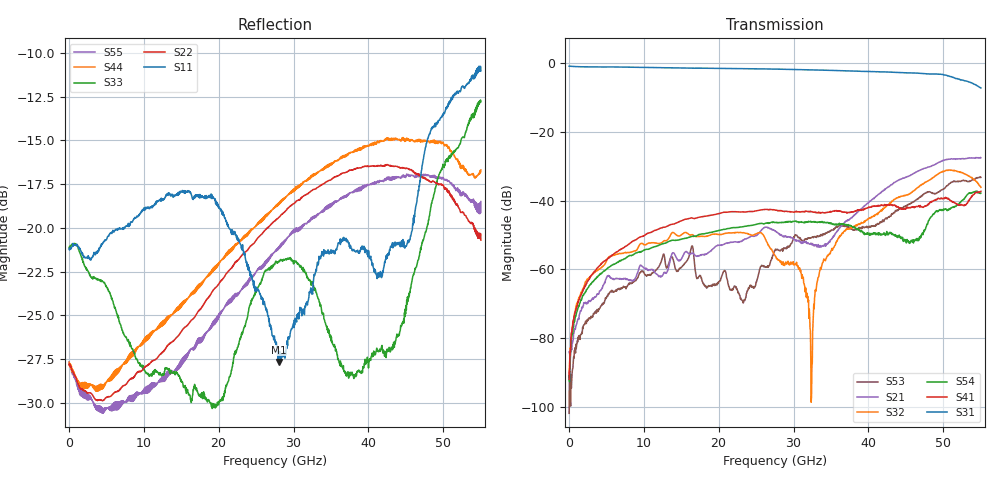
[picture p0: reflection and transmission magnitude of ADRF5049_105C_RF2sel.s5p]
! Device  : ADRF5049
! Description: Silicon SP4T Switch Non-Reflective
! Frequency:  9kHz -  45 GHz
! Ports:
!  RFC = Port 1
!  RF1 = Port 2
!  RF2 = Port 3
!	 RF3 = Port 4
!  RF4 = Port 5
! VSS  =  +3.30 Volts
! VDD  =  -3.30 Volts
! EN  =  0.00 Volts
! LS  =  0.00 Volts
! V1  =  3.30 Volts
! V2  =  0.00 Volts
! Data:  Data was collected using an calibrated 4 port network analyzer.
! Notes: Analog Devices supplies this data as a sample of measured data
!  for this product.  Your particular data for this product may vary.
!  Data was taken at 105 degrees C.
!  Analog Devices reserves the right to change this data at anytime.
# hz S db R 50
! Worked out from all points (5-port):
!   1100 points, 50 MHz to 55 GHz, reference 50 ohm
!   strongest paths, dB at 50 MHz, 13.8 GHz, 27.55 GHz, 41.3 GHz, 55 GHz:
!     S31: -0.9, -1.4, -1.7, -2.5, -7.2
!     S41: -92.0, -46.9, -42.7, -41.4, -37.3
!     S54: -90.9, -51.6, -46.4, -49.4, -37.8
!     S32: -91.1, -49.3, -56.1, -43.8, -36.1
!     S21: -84.1, -55.4, -49.0, -38.2, -27.5
!     S53: -101.9, -56.5, -54.2, -46.7, -33.2
!   lowest |S11| = -27.7 dB at 28 GHz (marker M1), VSWR 1.09, Z = 52.6 - j3.33 ohm
!   |S11| at or under -10 dB: start of sweep to end of sweep
